(* Logix 5000 AddOnInstructionDefinition export i550_Protec_Actuator_Speed; software revision 20.01 *)

ADD_ON_INSTRUCTION i550_Protec_Actuator_Speed   (* revision 1.1 *)
// Basic speed control for an i550 Protec drive
// Revision note:
// For use with EDS file Lenze_IOFW55AGXX_V4-20191120
VAR_IN_OUT
   i500_Drive_Control_Output : _024B:2019_11_20_i550_Prote_6E728D0C:O:0; {required}
   i500_Drive_State_Input : _024B:2019_11_20_i550_Prote_EDB64C9E:I:0; {required}
END_VAR
VAR_INPUT
   xEnableDrive : BOOL;   // Enable i550 drive
   xResetError : BOOL;   // Reset Drive Error
   xSetQuickStop : BOOL;   // Ramp down to 0 RPM using Quick Stop Decel. Time (0x291C or P225)
   xEnableVelocity : BOOL; {access None}   // Enable velocity control
   xInvertDirection : BOOL; {access None}   // Change motor Direction. 0 = Positive, 1 = Negative
   iSetVelocity : INT; {access None}   // Set Velocity in RPM
END_VAR
VAR_OUTPUT
   xAxisReady : BOOL; {access Read Only}   // Drive is ready
   xDriveWarning : BOOL; {access None}   // Drive warning active
   xAxisEnabled : BOOL; {access None}   // Drive is enabled
   xDriveError : BOOL; {access None}   // Drive error active
   diDriveErrorID : DINT; {access None}   // Error Code
   xDriveQspActive : BOOL; {access None}   // Quickstop is active (ramp to 0 RPM)
   iActualVelocity : INT; {access None}   // Current velocity in RPM
   xDirectionPositive : BOOL; {access None}   // Positive Direction active
   xDirectionNegative : BOOL; {access None}   // Negative direction active
   xSpeedEqZero : BOOL; {access None}   // When speed is zero
END_VAR
VAR
   siProfileState : SINT; {access None}
END_VAR

ROUTINE Logic   (* structured text *)
   //Initialize Output variables
   xAxisEnabled:=0;
   xDriveQspActive:=0;
   
   //Assign Inputs to control word
   i500_Drive_Control_Output.Data[0].0		:= not xInvertDirection and xEnableDrive; //Run Fwd
   i500_Drive_Control_Output.Data[0].1		:= xInvertDirection and xEnableDrive; //Run Rev
   i500_Drive_Control_Output.Data[0].2		:= xResetError; 				//Fault Reset
   i500_Drive_Control_Output.Data[0].5		:= 1; 							//Network Control (Enable)
   i500_Drive_Control_Output.Data[0].6		:= 1; 							//Network Speed Reference (Enable)
   i500_Drive_Control_Output.Data[0].12	:= not xEnableDrive;			//inhibit
   i500_Drive_Control_Output.Data[0].13	:= xSetQuickStop;				//QSP
   i500_Drive_Control_Output.Data[0].14	:= xSpeedEqZero;				//PID Off
   //i500_Drive_Control_Output.Data[0].15	:= ;							//DC Brake
   
   if xEnableVelocity then
   	i500_Drive_Control_Output.Data[1]:=iSetVelocity;
   else
   	i500_Drive_Control_Output.Data[1]:=0;
   end_if;
   
   // convert profile state, 1:Startup,2:Not_Ready,3:Ready,4:Enabled,5:Stopping,6:Fault_Stop,7:Faulted
   siProfileState.0:=i500_Drive_State_Input.Data[0].8;
   siProfileState.1:=i500_Drive_State_Input.Data[0].9;
   siProfileState.2:=i500_Drive_State_Input.Data[0].10;
   siProfileState.3:=i500_Drive_State_Input.Data[0].11;
   
   //check enable status
   if siProfileState = 4 then
   	xAxisEnabled:=1;
   end_if;
   
   //check quickstop status
   if xSetQuickStop and siProfileState = 5 then
   	xDriveQspActive:=1;
   end_if;
   
   //direct assignments of outputs
   xDriveError			:=i500_Drive_State_Input.Data[0].0;
   xDriveWarning		:=i500_Drive_State_Input.Data[0].1;
   xDirectionPositive	:=i500_Drive_State_Input.Data[0].2;
   xDirectionNegative	:=i500_Drive_State_Input.Data[0].3;
   xAxisReady			:=i500_Drive_State_Input.Data[0].4;
   iActualVelocity		:=i500_Drive_State_Input.Data[1];
   diDriveErrorID		:=i500_Drive_State_Input.Data[3];
   
   if iActualVelocity = 0 then
   xSpeedEqZero := 1;
   else;
   xSpeedEqZero := 0;
   end_if;
END_ROUTINE
END_ADD_ON_INSTRUCTION
